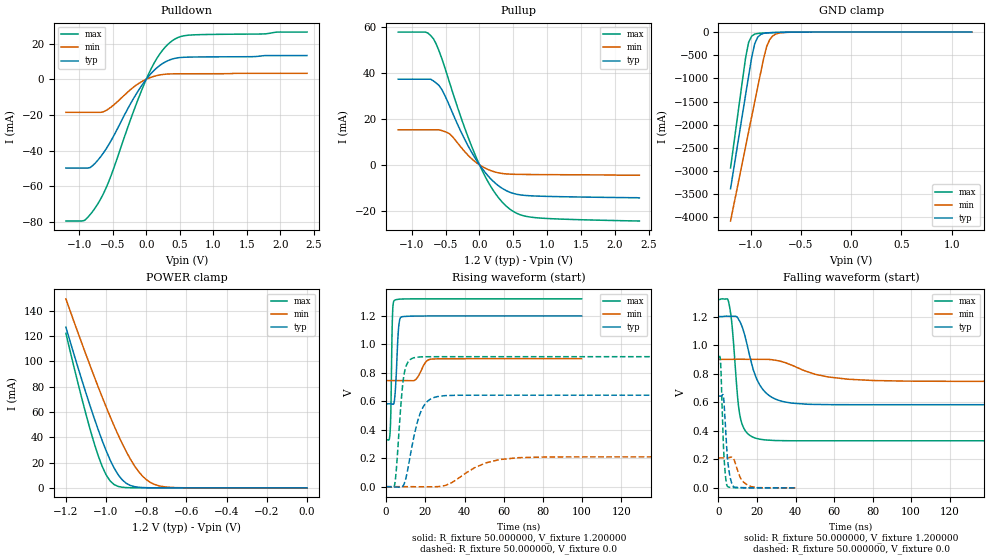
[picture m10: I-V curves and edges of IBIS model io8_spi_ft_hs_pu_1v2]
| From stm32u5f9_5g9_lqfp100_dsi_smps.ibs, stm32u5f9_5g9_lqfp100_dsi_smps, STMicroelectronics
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|   Model io8_spi_ft_hs_pu_1v2
[Model]  io8_spi_ft_hs_pu_1v2
Model_type I/O
Polarity   Non-Inverting
Enable   Active-Low
Vinl =   0.360000V
Vinh =   0.840000V
Vmeas =  0.600000V
Cref =   50.000000pF
Rref =   100.000000M
Vref =   0.0V
C_comp   3.132800pF   3.069700pF   3.178000pF
[Temperature Range]   25.000000   0.140000k   -40.000000
[Pullup Reference]   1.200000V   0.900000V   1.320000V
[Pulldown Reference]   0.0V   0.0V   0.0V
[POWER Clamp Reference]   1.200000V   0.900000V   1.320000V
[GND Clamp Reference]   0.0V   0.0V   0.0V
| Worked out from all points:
|   slope of the pulldown table from 0 to 0.18 V, typ, clamps not added: 25.4 ohm
|   slope of the pullup table from 0 to 0.18 V, typ, clamps not added: 27.8 ohm
|   GND clamp passes 1 mA (typ) near -0.51 V on its own axis
|   POWER clamp passes 1 mA (typ) near -0.86 V on its own axis
|   rising waveform, R_fixture 50.000000, V_fixture 1.200000: 20-80 % time 1.31ns typ, 3.46ns min, 670ps max; typ from 0.583 V to 1.2 V
|   rising waveform, R_fixture 50.000000, V_fixture 0.0: 20-80 % time 6.23ns typ, 16ns min, 3.02ns max; typ from 0 V to 0.643 V
|   falling waveform, R_fixture 50.000000, V_fixture 1.200000: 20-80 % time 8.69ns typ, 20.8ns min, 3.71ns max; typ from 1.2 V to 0.583 V
|   falling waveform, R_fixture 50.000000, V_fixture 0.0: 20-80 % time 2.11ns typ, 4.03ns min, 1.52ns max; typ from 0.643 V to 0 V
[Pulldown]
|Voltage   I(typ)   I(min)   I(max)
-1.2V     -49.85mA   -18.57mA   -79.56mA
-920mV    -49.85mA   -18.57mA   -79.19mA
-840mV    -49.59mA   -18.57mA   -76.08mA
-720mV    -45.32mA   -18.57mA   -69.73mA
-560mV    -36.71mA   -16.58mA   -57.44mA
-200mV    -11.43mA   -4.74mA    -19.03mA
0V        0A         0A         0A
160mV     6.476mA    2.075mA    11.78mA
360mV     10.99mA    2.989mA    20.81mA
480mV     12.07mA    3.053mA    23.52mA
640mV     12.42mA    3.074mA    24.76mA
2.4V      13.3mA     3.331mA    26.5mA
[Pullup]
|Voltage   I(typ)   I(min)   I(max)
-1.2V     37.31mA    15.26mA    57.87mA
-800mV    37.31mA    15.26mA    57.87mA
-680mV    36.57mA    15.26mA    54.97mA
-560mV    33mA       15mA       46.62mA
-440mV    25.52mA    13.49mA    35.66mA
-200mV    10.05mA    5.175mA    14.59mA
0V        580fA      233pA      0A
200mV     -7.072mA   -2.851mA   -11mA
440mV     -11.84mA   -4.03mA    -19.1mA
600mV     -13.07mA   -4.154mA   -21.71mA
840mV     -13.59mA   -4.223mA   -23.04mA
2.36V     -14.4mA    -4.5mA     -24.46mA
[GND_clamp]
|Voltage   I(typ)   I(min)   I(max)
-1.2V     -3.379A    -4.076A    -2.932A
-1.05V    -1.35A     -2.47A     -550.7mA
-1.02V    -947.8mA   -2.149A    -221.5mA
-990mV    -552.4mA   -1.829A    -88.44mA
-960mV    -255.3mA   -1.51A     -44.87mA
-930mV    -111.8mA   -1.191A    -30.68mA
-870mV    -28.35mA   -564.6mA   -21.34mA
-840mV    -18.65mA   -309.5mA   -18.49mA
-810mV    -14.07mA   -161.6mA   -15.92mA
-780mV    -11.37mA   -83.33mA   -13.53mA
-600mV    -3.009mA   -4.321mA   -3.091mA
1.2V      0A         13.65nA    0A
[POWER_clamp]
|Voltage   I(typ)   I(min)   I(max)
-1.2V     127mA      149.4mA    122.2mA
-1.12V    84.98mA    114mA      70.29mA
-1.06V    55.52mA    88.42mA    35.69mA
-1.02V    37.64mA    72.04mA    17.19mA
-1V       29.52mA    64.13mA    10.33mA
-960mV    15.7mA     48.99mA    2.596mA
-900mV    3.636mA    28.77mA    207.8uA
-840mV    502.9uA    13.24mA    43.56uA
-800mV    129uA      6.535mA    43.56uA
-740mV    25.5uA     1.726mA    43.56uA
-620mV    25.17uA    82.33uA    36.07uA
0V        0A         17.36nA    0A
[Ramp]
| variable   typ   min   max
dV/dt_r  0.38569/6.22410n   0.12565/15.93205n   0.54819/3.00537n
dV/dt_f  0.37036/8.68183n   92.33400m/20.75663n 0.59402/3.70384n
R_load = 50.000000
[Rising Waveform]
R_fixture= 50.000000
V_fixture= 1.200000
V_fixture_min= 0.900000
V_fixture_max= 1.320000
|time   V(typ)   V(min)   V(max)
0s        582.7mV    746.1mV    330mV
2.002ns   582.8mV    746.1mV    380.9mV
2.402ns   582.7mV    746.1mV    526.6mV
3.203ns   580.7mV    746.1mV    1.195V
4.204ns   604.7mV    746.1mV    1.309V
6.406ns   1.125V     746.1mV    1.317V
7.808ns   1.193V     746.1mV    1.319V
14.81ns   1.199V     750.3mV    1.32V
23.02ns   1.2V       896.6mV    1.32V
99.7ns    1.2V       900mV      1.32V
[Rising Waveform]
R_fixture= 50.000000
V_fixture= 0.0
V_fixture_min= 0.0
V_fixture_max= 0.0
|time   V(typ)   V(min)   V(max)
0s        435.5uV    496.6uV    378.9uV
4.404ns   -1.414mV   496.4uV    18.61mV
8.809ns   9.48mV     495.4uV    760.2mV
10.81ns   107.4mV    504.4uV    867.5mV
14.01ns   343.7mV    353.3uV    905.5mV
19.22ns   568.4mV    -527.5uV   913mV
27.23ns   635.9mV    2.081mV    913.7mV
50.85ns   643.2mV    167.6mV    913.7mV
67.67ns   643.2mV    204.3mV    913.7mV
199.4ns   643.3mV    210mV      913.8mV
[Falling Waveform]
R_fixture= 50.000000
V_fixture= 1.200000
V_fixture_min= 0.900000
V_fixture_max= 1.320000
|time   V(typ)   V(min)   V(max)
0s        1.2V       900mV      1.32V
5.205ns   1.202V     899.9mV    1.304V
6.807ns   1.202V     900mV      1.169V
10.01ns   1.19V      901.1mV    622.7mV
11.21ns   1.162V     901.1mV    500.6mV
18.82ns   798.9mV    900.6mV    350.5mV
26.03ns   649.8mV    899.9mV    334.5mV
38.44ns   593.3mV    857.4mV    330.1mV
67.67ns   582.9mV    760.8mV    330mV
199.4ns   582.7mV    746.1mV    330mV
[Falling Waveform]
R_fixture= 50.000000
V_fixture= 0.0
V_fixture_min= 0.0
V_fixture_max= 0.0
|time   V(typ)   V(min)   V(max)
0s        643.3mV    210mV      913.8mV
1.121ns   642.9mV    210mV      870mV
2.563ns   641.4mV    210mV      298.2mV
3.524ns   453.9mV    209.9mV    98mV
4.565ns   225.9mV    209.9mV    12.4mV
6.166ns   66.99mV    214.3mV    3.646mV
7.848ns   7.875mV    204.1mV    1.758mV
11.61ns   2.285mV    65.13mV    781.6uV
15.54ns   1.157mV    17.19mV    539.8uV
39.88ns   435.5uV    496.6uV    378.9uV
